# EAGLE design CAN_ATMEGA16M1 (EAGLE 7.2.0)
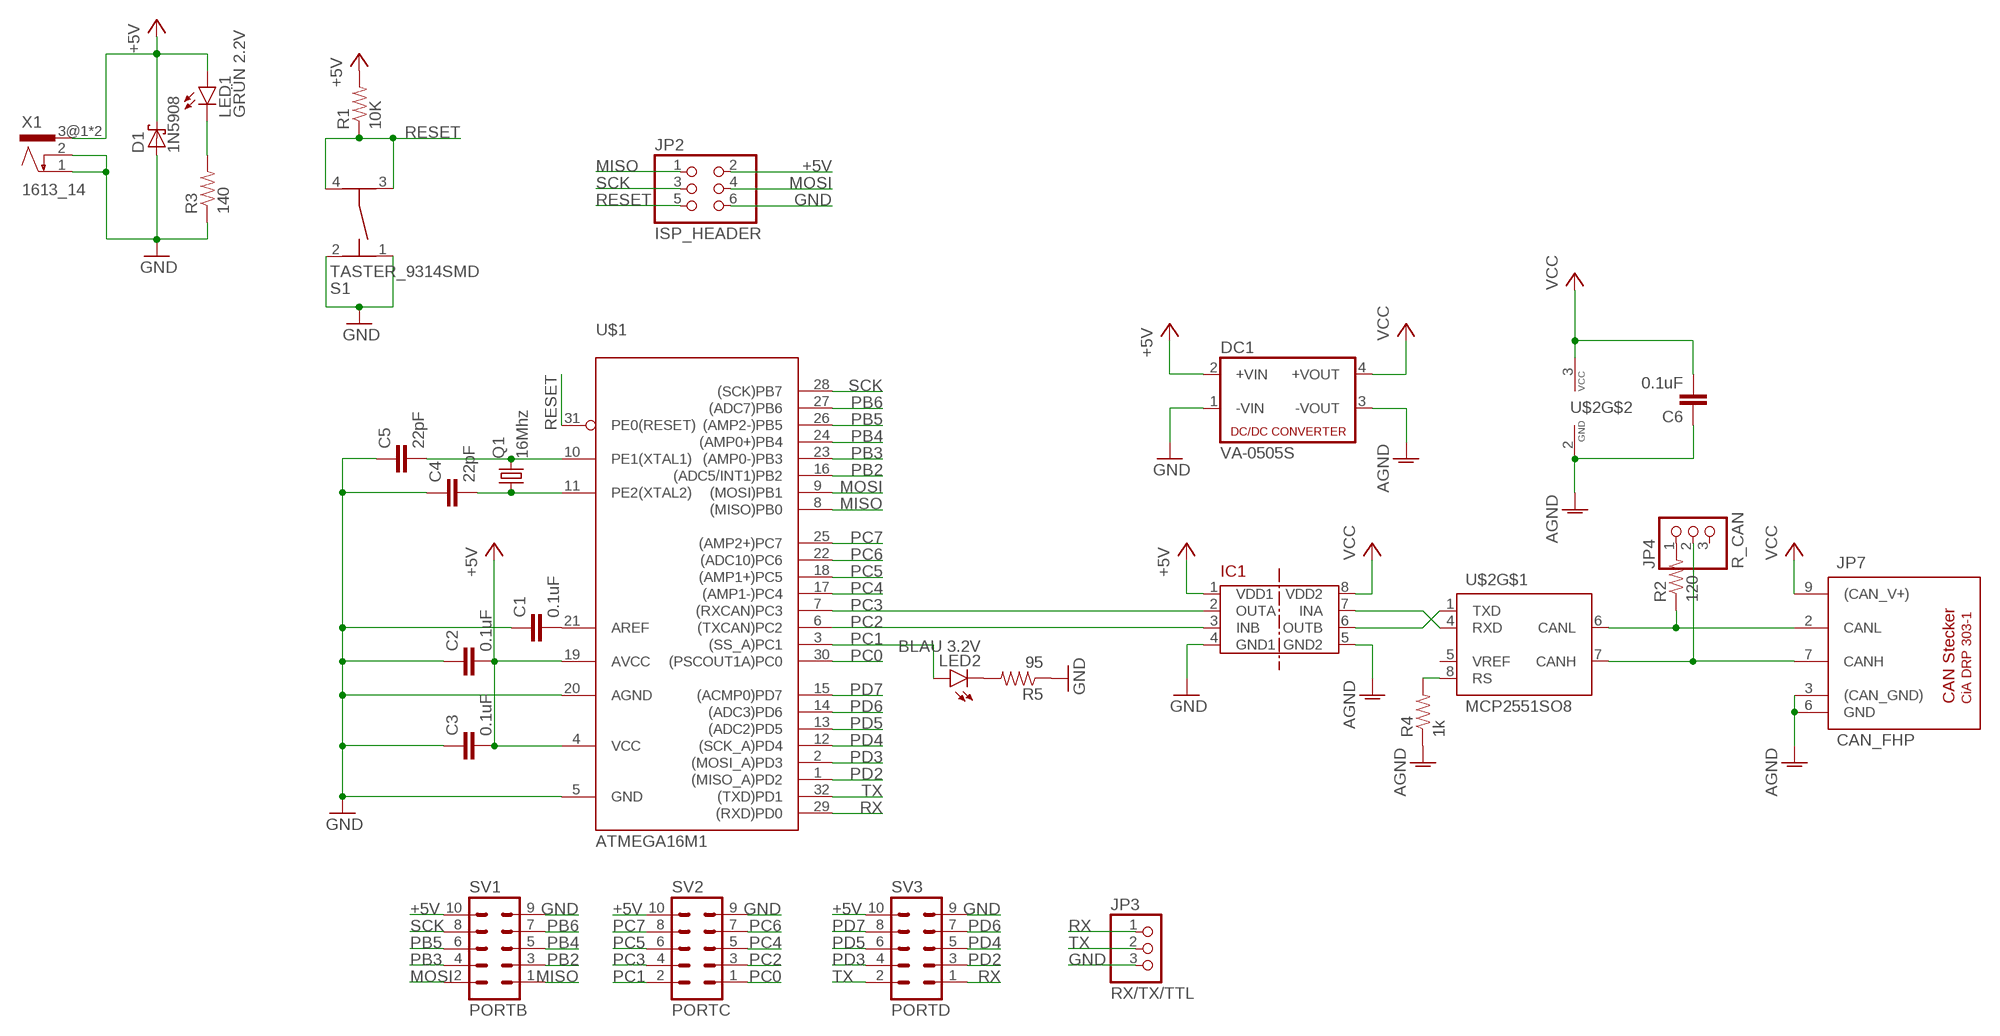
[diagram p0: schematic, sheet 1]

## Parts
C1  0.1uF  0.1UF-25V(+80/-20%)(0603)  [0603-CAP]
C2  0.1uF  0.1UF-25V(+80/-20%)(0603)  [0603-CAP]
C3  0.1uF  0.1UF-25V(+80/-20%)(0603)  [0603-CAP]
C4  22pF  0.1UF-25V(+80/-20%)(0603)  [0603-CAP]
C5  22pF  0.1UF-25V(+80/-20%)(0603)  [0603-CAP]
C6  0.1uF  0.1UF-25V(+80/-20%)(0603)  [0603-CAP]
D1  1N5908  [C4111-15]
DC1  VA-0505S  [4SIL]
IC1  ADUM1201  [SO8]
JP2  ISP_HEADER  PINHD-2X3  [2X03]
JP3  RX/TX/TTL  PINHD-1X3  [1X03]
JP4  R_CAN  PINHD-1X3  [1X03]
JP7  CAN_FHP  [F09HP]
LED1  GRÜN 2.2V  LED-FKIT-1206  [FKIT-LED-1206]
LED2  BLAU 3.2V  LED-FKIT-1206  [FKIT-LED-1206]
Q1  16Mhz  CRYSTALHC49UP  [HC49UP]
R1  10K  10KOHM-1/10W-1%(0603)0603  [0603-RES]
R2  120  10KOHM-1/10W-1%(0603)0603  [0603-RES]
R3  140  10KOHM-1/10W-1%(0603)0603  [0603-RES]
R4  1k  10KOHM-1/10W-1%(0603)0603  [0603-RES]
R5  95  10KOHM-1/10W-1%(0603)0603  [0603-RES]
S1  TASTER_9314SMD  [TASTER_9314SMD]
SV1  PORTB  ML10  [ML10]
SV2  PORTC  ML10  [ML10]
SV3  PORTD  ML10  [ML10]
U$1  ATMEGA16M1  [TQFP32]
U$2  MCP2551SO8  [SO08]
X1  1613_14  [1613_14]

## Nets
+5V: C2.2 C3.2 D1.C DC1.2(+VIN) IC1.1(VDD1) JP2.2 LED1.A R1.2 SV1.10 SV2.10 SV3.10 U$1.4(VCC) U$1.19(AVCC) X1.3@1 X1.3@2
AGND: C6.1 DC1.3(-VOUT) IC1.5(GND2) JP7.3((CAN_GND)) JP7.6(GND) R4.1 U$2.2(GND)
GND: C1.1 C2.1 C3.1 C4.1 C5.1 D1.A DC1.1(-VIN) IC1.4(GND1) JP2.6 JP3.3 R3.1 R5.1 S1.1 S1.2 SV1.9 SV2.9 SV3.9 U$1.5(GND) U$1.20(AGND) X1.1 X1.2
MISO: JP2.1 SV1.1 U$1.8((MISO)PB0)
MOSI: JP2.4 SV1.2 U$1.9((MOSI)PB1)
N$1: C1.2 U$1.21(AREF)
N$2: LED2.C R5.2
N$3: C4.2 Q1.1 U$1.11(PE2(XTAL2))
N$4: C5.2 Q1.2 U$1.10(PE1(XTAL1))
N$5: JP4.1 R2.2
N$8: JP7.2(CANL) R2.1 U$2.6(CANL)
N$9: JP4.2 JP7.7(CANH) U$2.7(CANH)
N$10: IC1.7(INA) U$2.4(RXD)
N$16: IC1.6(OUTB) U$2.1(TXD)
N$29: LED1.C R3.2
N$30: R4.2 U$2.8(RS)
PB2: SV1.3 U$1.16((ADC5/INT1)PB2)
PB3: SV1.4 U$1.23((AMP0-)PB3)
PB4: SV1.5 U$1.24((AMP0+)PB4)
PB5: SV1.6 U$1.26((AMP2-)PB5)
PB6: SV1.7 U$1.27((ADC7)PB6)
PC0: SV2.1 U$1.30((PSCOUT1A)PC0)
PC1: LED2.A SV2.2 U$1.3((SS_A)PC1)
PC2: IC1.3(INB) SV2.3 U$1.6((TXCAN)PC2)
PC3: IC1.2(OUTA) SV2.4 U$1.7((RXCAN)PC3)
PC4: SV2.5 U$1.17((AMP1-)PC4)
PC5: SV2.6 U$1.18((AMP1+)PC5)
PC6: SV2.7 U$1.22((ADC10)PC6)
PC7: SV2.8 U$1.25((AMP2+)PC7)
PD2: SV3.3 U$1.1((MISO_A)PD2)
PD3: SV3.4 U$1.2((MOSI_A)PD3)
PD4: SV3.5 U$1.12((SCK_A)PD4)
PD5: SV3.6 U$1.13((ADC2)PD5)
PD6: SV3.7 U$1.14((ADC3)PD6)
PD7: SV3.8 U$1.15((ACMP0)PD7)
RESET: JP2.5 R1.1 S1.3 S1.4 U$1.31(PE0(RESET))
RX: JP3.1 SV3.1 U$1.29((RXD)PD0)
SCK: JP2.3 SV1.8 U$1.28((SCK)PB7)
TX: JP3.2 SV3.2 U$1.32((TXD)PD1)
VCC: C6.2 DC1.4(+VOUT) IC1.8(VDD2) JP7.9((CAN_V+)) U$2.3(VCC)
Unconnected: JP4.3 U$2.5(VREF)

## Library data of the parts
C1-C3 C6 = SparkFun-Capacitors:0.1UF-25V(+80/-20%)(0603): CAP-00810; PROD_ID: CAP-00810
C4 C5 = SparkFun-Capacitors:0.1UF-25V(+80/-20%)(0603): CAP-00810; PROD_ID: CAP-00810; VALUE: 0.1uF
D1 = diode:1N5908: DIODE
DC1 = dc-dc-converter:VA-*?: DC DC Converter Single Output, 1 Watt Motien Technology Co.,Ltd. Source: Data sheet; OC_FARNELL: unknown; OC_NEWARK: unknown
IC1 = Bus-isolators:ADUM1201
JP2 = pinhead:PINHD-2X3: PIN HEADER
JP3 JP4 = pinhead:PINHD-1X3: PIN HEADER
JP7 = can:CAN_: CAN Stecker nach CiA DRP 303-1
LED1 LED2 = SparkFun-LED:LED: LEDs
Q1 = crystal:CRYSTAL: CRYSTAL; OC_FARNELL: unknown; OC_NEWARK: unknown
R1 = SparkFun-Resistors:10KOHM-1/10W-1%(0603): RES-00824; PROD_ID: RES-00824
R2-R5 = SparkFun-Resistors:10KOHM-1/10W-1%(0603): RES-00824; PROD_ID: RES-00824; VALUE: 10K
S1 = EmbeddedProjectsBauteile:TASTER_9314SMD: Taster Würth Elektronik
SV1-SV3 = con-harting-ml:ML10: HARTING; OC_FARNELL: unknown; OC_NEWARK: unknown
U$1 = EmbeddedProjectsBauteile:ATMEGA16M1: Atmel Low Power AVR 8-bit Microcontroller 16K with CAN; EP: 40880
U$2 = can:MCP2551: CAN Tranceiver Microchip
X1 = con-lumberg:1613_14: Power supply connectors / Netzgeräte-Steckverbinder Source: Data sheet; MF: LUMBERG; MPN: 1613 14; OC_FARNELL: 1243245

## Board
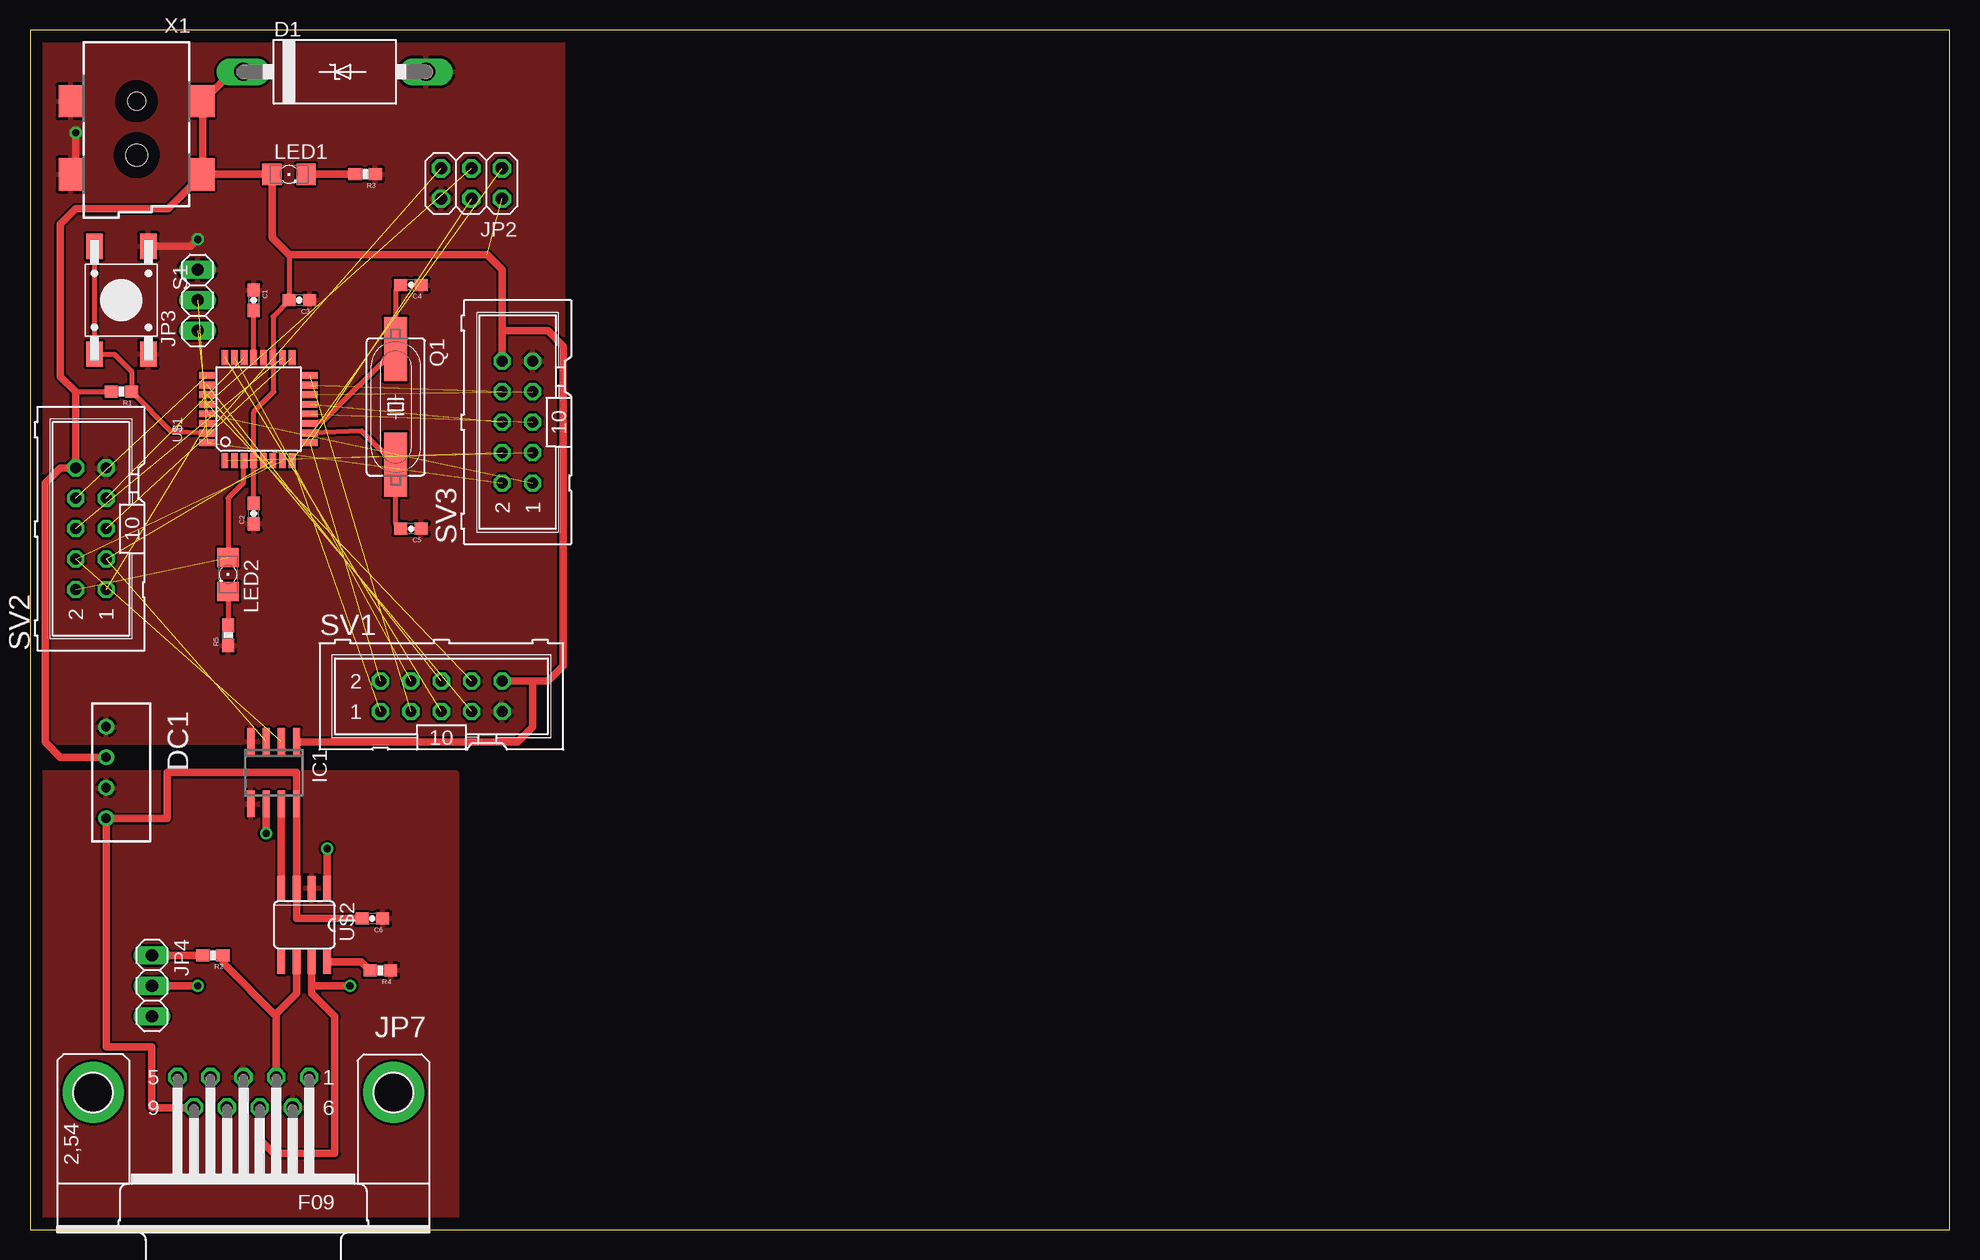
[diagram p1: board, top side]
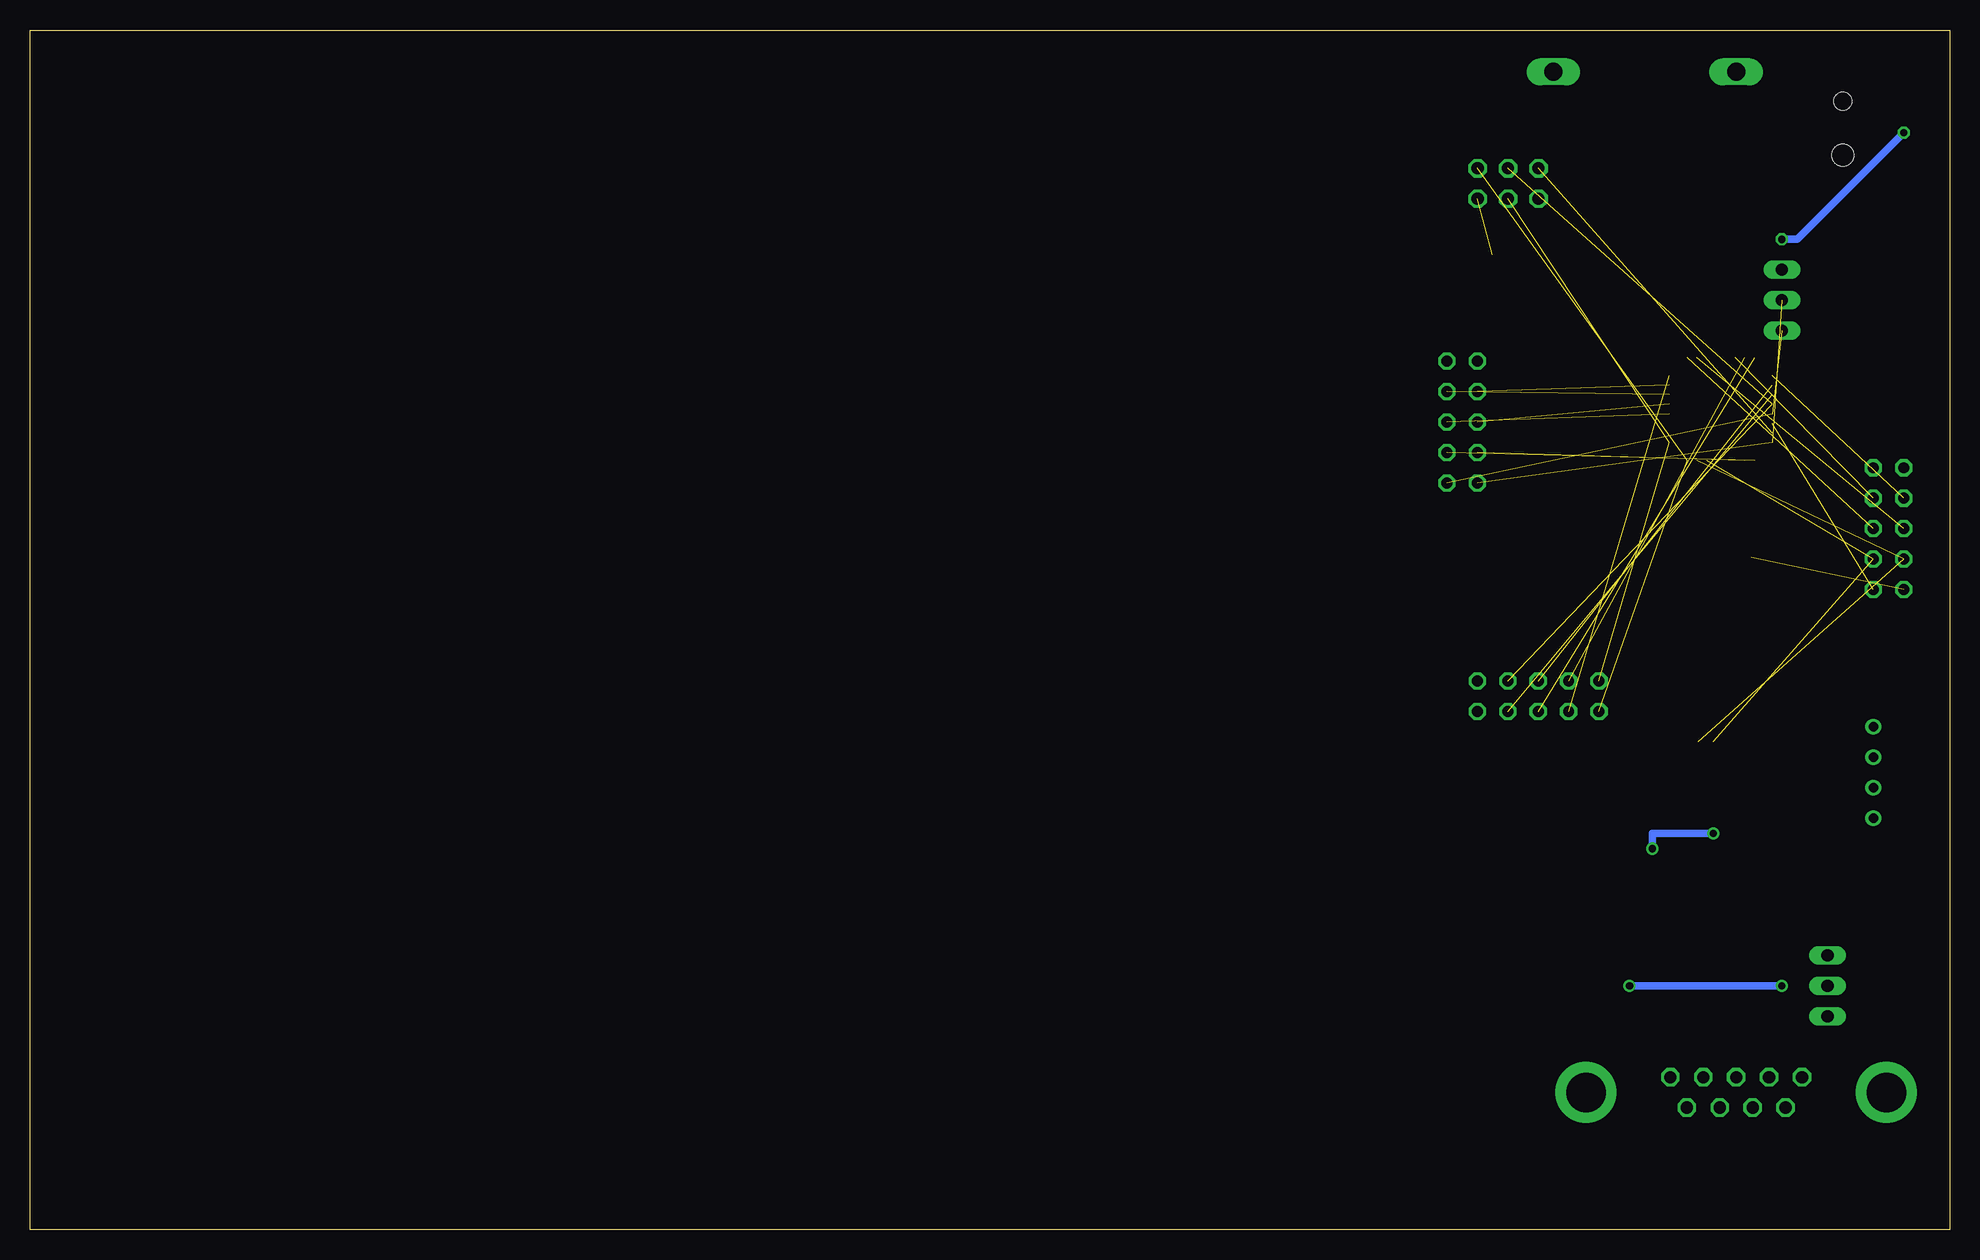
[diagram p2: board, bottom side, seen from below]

Size 160 x 100 mm. Coordinates in mm from the lower left corner, seen from the top.
Outline: 0,0 160,0 160,100 0,100 0,0
Copper layers (1*16): Top 0.035mm / dielectric 1.5mm / Bottom 0.035mm
Design rules "default": minimum track width 10mil, minimum drill 24mil, track to track 8mil, track to pad 8mil, pad to pad 8mil, via to via 8mil, smd to smd 8mil, copper to edge 40mil, drill to drill 8mil, minimum pad ring 10mil, minimum via ring 8mil, stop-mask expansion 4mil, vias tented up to drill 0mil, thermal gap 10mil

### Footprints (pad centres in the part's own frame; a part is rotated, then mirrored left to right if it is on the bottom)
0603-CAP = smd 1.1 x 1: 1 -0.85,0; 2 0.85,0
C4111-15 = drill 1.499 long: A 7.62,0; C -7.62,0
4SIL = drill 0.8: 1 -3.81,0; 2 -1.27,0; 3 1.27,0; 4 3.81,0
SO8 = smd 0.6 x 2.2: 1 -1.905,-2.6; 2 -0.635,-2.6; 3 0.635,-2.6; 4 1.905,-2.6; 5 1.905,2.6; 6 0.635,2.6; 7 -0.635,2.6; 8 -1.905,2.6
2X03 = drill 1.016 octagon: 1 -2.54,-1.27; 2 -2.54,1.27; 3 0,-1.27; 4 0,1.27; 5 2.54,-1.27; 6 2.54,1.27
1X03 = drill 1.016 long: 1 -2.54,0; 2 0,0; 3 2.54,0
F09HP = drill 1.016 octagon: 1 -5.486,-1.27; 2 -2.743,-1.27; 3 0,-1.27; 4 2.743,-1.27; 5 5.486,-1.27; 6 -4.115,1.27; 7 -1.372,1.27; 8 1.372,1.27; 9 4.115,1.27 | drill 3.302 pad 5.08: G1 -12.522,0; G2 12.522,0
FKIT-LED-1206 = smd 1.6 x 1.803: A -1.422,0; C 1.422,0
HC49UP = smd 5.334 x 1.93: 1 -4.826,0; 2 4.826,0
0603-RES = smd 1.1 x 1: 1 -0.85,0; 2 0.85,0
TASTER_9314SMD = smd 2.1 x 1.4: 1 -4.492,2.25; 2 4.492,2.25; 3 -4.492,-2.25; 4 4.492,-2.25
ML10 = drill 0.914 octagon: 1 -5.08,-1.27; 2 -5.08,1.27; 3 -2.54,-1.27; 4 -2.54,1.27; 5 0,-1.27; 6 0,1.27; 7 2.54,-1.27; 8 2.54,1.27; 9 5.08,-1.27; 10 5.08,1.27
TQFP32 = smd 1.27 x 0.559: 1 -4.293,2.8; 2 -4.293,2; 3 -4.293,1.2; 4 -4.293,0.4; 5 -4.293,-0.4; 6 -4.293,-1.2; 7 -4.293,-2; 8 -4.293,-2.8; 17 4.293,-2.8; 18 4.293,-2; 19 4.293,-1.2; 20 4.293,-0.4; 21 4.293,0.4; 22 4.293,1.2; 23 4.293,2; 24 4.293,2.8 | smd 0.559 x 1.27: 9 -2.8,-4.293; 10 -2,-4.293; 11 -1.2,-4.293; 12 -0.4,-4.293; 13 0.4,-4.293; 14 1.2,-4.293; 15 2,-4.293; 16 2.8,-4.293; 25 2.8,4.293; 26 2,4.293; 27 1.2,4.293; 28 0.4,4.293; 29 -0.4,4.293; 30 -1.2,4.293; 31 -2,4.293; 32 -2.8,4.293
SO08 = smd 0.66 x 2.032: 1 -1.905,-3.073; 2 -0.635,-3.073; 3 0.635,-3.073; 4 1.905,-3.073; 5 1.905,3.073; 6 0.635,3.073; 7 -0.635,3.073; 8 -1.905,3.073
1613_14 = smd 2 x 2.7: 1 5.5,5; 2 5.5,11.1; 3@1 -5.5,11.1; 3@2 -5.5,5 | hole 1.5: 0,5 | hole 1.8: 0,9.5

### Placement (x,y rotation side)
C1  18.65,77.47 270 top
C2  18.65,59.69 90 top
C3  22.45,77.47 180 top
C4  31.75,78.74 180 top
C5  31.75,58.42 180 top
C6  28.54,25.92 180 top
D1  25.4,96.52 0 top
DC1  6.35,38.1 270 top
IC1  20.32,38.1 180 top
JP2  36.8,87.2 180 top
JP3  13.97,77.47 90 top
JP4  10.16,20.32 270 top
JP7  17.78,11.43 180 top
LED1  21.59,87.97 0 top
LED2  16.51,54.61 270 top
Q1  30.48,68.58 270 top
R1  7.62,69.85 180 top
R2  15.24,22.86 180 top
R3  27.94,87.97 180 top
R4  29.21,21.59 180 top
R5  16.51,49.53 90 top
S1  7.62,77.47 270 top
SV1  34.29,44.45 0 top
SV2  5.08,58.42 90 top
SV3  40.64,67.31 90 top
U$1  19.05,68.4 90 top
U$2  22.86,25.4 180 top
X1  8.89,99.06 180 top

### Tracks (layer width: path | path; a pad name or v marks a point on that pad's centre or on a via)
+5V  (1 unrouted)
  Top 0.406: 21.59,81.28 C3.2 20.25,76.12 U$1.19 20.32,72.8 20.32,69.85 18.65,68.18 U$1.4 C2.2 | 3.81,69.85 R1.2
  Top 0.61: D1.C 16.85,96.52 X1.3@2 X1.3@1 | X1.3@1 LED1.A 20.17,82.7 21.59,81.28 38.1,81.28 39.37,80.01 39.37,74.93 | 39.37,74.93 SV3.10 | X1.3@1 11.52,85.09 3.81,85.09 2.54,83.82 2.54,71.12 3.81,69.85 SV2.10 2.54,63.5 1.27,62.23 1.27,40.64 2.54,39.37 DC1.2 | SV1.10 41.91,45.72 | 41.91,45.72 43.18,45.72 44.45,46.99 44.45,73.66 43.18,74.93 39.37,74.93 | IC1.1 22.29,40.64 40.64,40.64 41.91,41.91 41.91,45.72
AGND
  pour Top: 0,0 0,38.1 35.56,38.1 35.56,0
GND  (via drill 0.6)
  Top 0.61: X1.2 3.81,88.38 v3.81,91.44 | v13.97,82.55 13.38,81.96 S1.1
  Bottom 0.61: v3.81,91.44 12.7,82.55 v13.97,82.55
  pour Top: 0,100.33 0,40.64 44.45,40.64 44.45,100.33
MISO  (2 unrouted)
MOSI  (2 unrouted)
N$1
  Top 0.406: U$1.21 C1.2
N$2
  Top 0.406: LED2.C R5.2
N$3
  Top 0.406: U$1.11 24.45,67.38 Q1.1 30.48,78.32 C4.2
N$4
  Top 0.406: U$1.10 27.65,66.58 Q1.2 30.48,58.84 C5.2
N$5
  Top 0.61: JP4.1 R2.2
N$8
  Top 0.61: JP7.2 20.52,17.78 | 20.52,17.78 20.52,17.98 22.23,19.68 U$2.6 | R2.1 16.09,22.21 20.52,17.78
N$9  (via drill 0.6)
  Top 0.61: JP7.7 19.15,7.52 20.32,6.35 25.4,6.35 25.4,17.78 23.5,19.68 23.5,20.32 | 23.5,20.32 U$2.7 | JP4.2 v13.97,20.32 | v26.67,20.32 23.5,20.32
  Bottom 0.61: v13.97,20.32 v26.67,20.32
N$10
  Top 0.61: IC1.7 U$2.4
N$16  (via drill 0.6)
  Top 0.61: IC1.6 v19.68,33.02 | v24.77,31.75 U$2.1
  Bottom 0.61: v19.68,33.02 24.77,33.02 v24.77,31.75
N$29
  Top 0.61: R3.2 LED1.C
N$30
  Top 0.61: U$2.8 27.62,22.33 R4.2
PB2  (1 unrouted)
PB3  (1 unrouted)
PB4  (1 unrouted)
PB5  (1 unrouted)
PB6  (1 unrouted)
PC0  (1 unrouted)
PC1  (1 unrouted)
  Top 0.406: U$1.3 17.78,64.22 17.78,62.23 16.51,60.96 LED2.A
PC2  (2 unrouted)
PC3  (2 unrouted)
PC4  (1 unrouted)
PC5  (1 unrouted)
PC6  (1 unrouted)
PC7  (1 unrouted)
PD2  (1 unrouted)
PD3  (1 unrouted)
PD4  (1 unrouted)
PD5  (1 unrouted)
PD6  (1 unrouted)
PD7  (1 unrouted)
RESET  (1 unrouted)
  Top 0.406: S1.3 S1.4 7.03,72.98 8.47,71.54 R1.1 11.74,66.58 U$1.31
RX  (2 unrouted)
SCK  (2 unrouted)
TX  (2 unrouted)
VCC
  Top 0.61: JP7.9 10.16,10.16 10.16,15.24 6.35,15.24 DC1.4 11.43,34.29 11.43,38.1 22.23,38.1 IC1.8 U$2.3 22.23,25.92 C6.2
